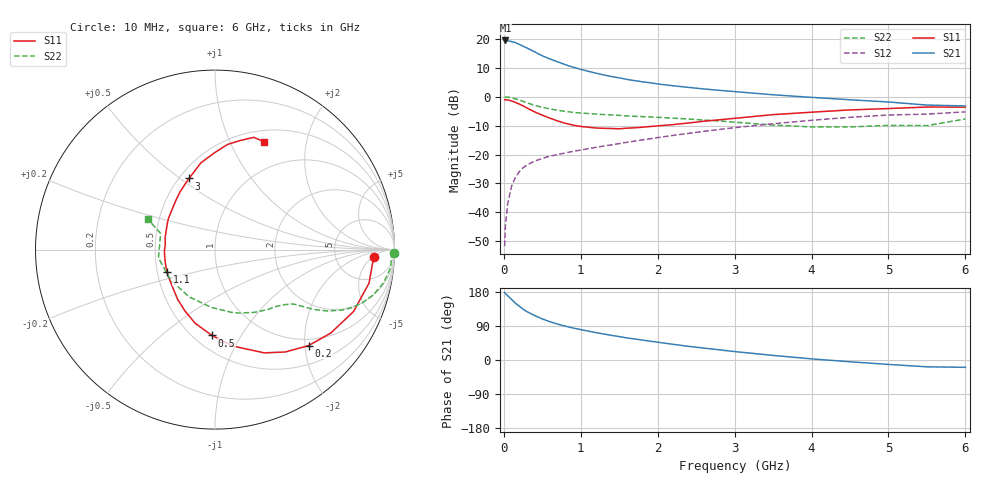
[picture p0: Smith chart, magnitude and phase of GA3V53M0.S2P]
! Infineon Technologies  Discrete & RF Semiconductors
! BF775
! Si NPN RF Bipolar Junction Transistor in SOT23
! VCE = 3.5 V  IC = 3 mA
! Common Emitter S-Parameters:  May  1996
# GHz  S  MA  R  50
!  f  S11  S21  S12  S22
! GHz  MAG  ANG  MAG  ANG  MAG  ANG  MAG  ANG
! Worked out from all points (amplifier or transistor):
!   36 points, 10 MHz to 6 GHz, reference 50 ohm
!   highest |S21| = 19.4 dB at 20 MHz (marker M1)
!   |S21| within 3 dB of that: start of sweep to 330.3 MHz
!   unconditionally stable (mu >= 1): 990.3 MHz to 3.538 GHz
!   at 250 MHz: K = 0.36, MSG = 21.0 dB, |S12| = -24.6 dB
!   at 1.4 GHz: K = 1.12, MAG = 9.7 dB, |S12| = -16.7 dB
!   at 6 GHz: K = 0.97, MSG = 1.0 dB, |S12| = -5.2 dB
!   S11 on the Smith chart (normalised r, x): 10 MHz: 15, -5; 200 MHz: 0.86, -2.08; 500 MHz: 0.61, -0.76; 1.1 GHz: 0.56, -0.16; 3 GHz: 0.56, +0.54; 6 GHz: 0.63, +1.35
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0.01  0.8876 -2.5  9.277 178.1  0.0026 87.5  0.997 -1.1
0.02  0.8809 -5.2  9.377 175.7  0.0058 87.3  0.9834 -2.3
0.05  0.8784 -12.3  9.31 169.7  0.0141 82.9  0.9847 -5.8
0.1  0.8454 -24.1  8.95 160.1  0.028 76.8  0.9578 -11.1
0.15  0.7951 -35.8  8.609 149.8  0.0402 70.9  0.9174 -16.0
0.2  0.747 -45.7  8.024 142.0  0.0504 65.7  0.8732 -19.8
0.25  0.6921 -55.5  7.46 134.3  0.0589 61.6  0.8299 -22.9
0.3  0.6375 -64.5  6.955 127.6  0.066 58.7  0.7858 -25.4
0.4  0.5458 -79.7  5.963 117.4  0.0769 54.2  0.7093 -28.8
0.5  0.4783 -92.1  5.086 108.3  0.0857 51.8  0.6539 -30.8
0.6  0.4248 -105.1  4.49 101.0  0.0935 50.2  0.6142 -32.0
0.7  0.3799 -116.3  4.003 94.7  0.1 50.0  0.5808 -33.0
0.8  0.3467 -126.8  3.574 89.2  0.1065 49.7  0.5554 -33.9
1.1  0.2961 -154.8  2.74 76.1  0.1264 50.3  0.51 -36.7
1.3  0.2834 -171.3  2.374 68.6  0.1404 50.9  0.4902 -38.9
1.6  0.2856 166.9  1.991 58.3  0.1626 51.4  0.4651 -42.9
2.2  0.3286 136.4  1.544 41.4  0.2138 50.5  0.425 -53.8
3  0.4221 110.0  1.223 22.2  0.2912 45.0  0.3621 -75.0
3.5  0.4893 99.3  1.079 12.1  0.3404 39.8  0.3226 -93.9
4.5  0.59 83.2  0.884 -4.7  0.4398 27.4  0.2997 -145.8
5.5  0.6619 70.9  0.716 -18.0  0.4991 11.9  0.3157 163.5
6  0.6599 65.6  0.691 -19.3  0.5464 7.6  0.4114 155.6
